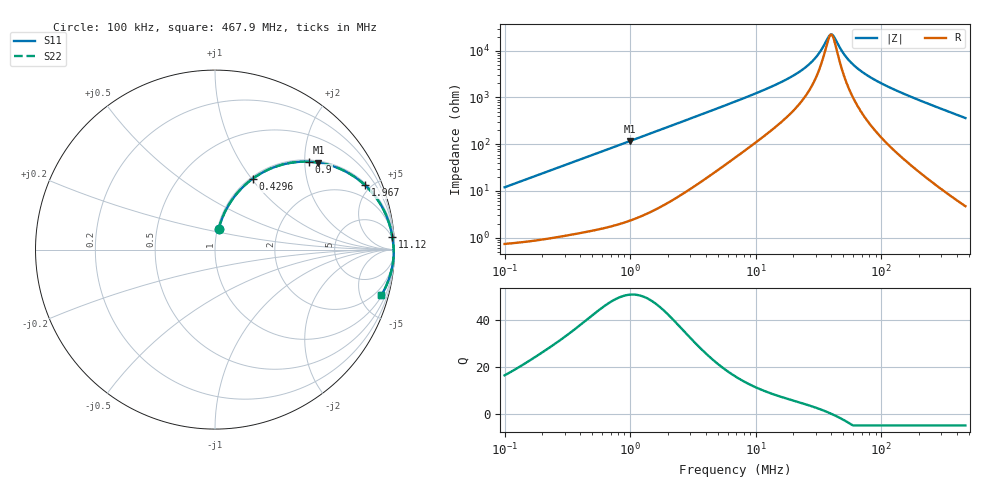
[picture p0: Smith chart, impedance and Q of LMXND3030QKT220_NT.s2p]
! LMXND3030QKT220_NT  S-PARAMETER MODEL  ( Standard Model )
! Model Generated by TAIYO YUDEN Corporation (https://www.yuden.co.jp/en/)
! Version 1.0
! TAIYO YUDEN Control No. 20250724
! Copyright(c) 2025 TAIYO YUDEN CO.,LTD. All Rights Reserved.
! Product Description (link to TY-COMPAS)
! https://ds.yuden.co.jp/TYCOMPAS/or/detail?pn=LMXND3030QKT220MNT&u=M
! Products Name : Inductors
! Characteristics :
!  Inductance : 22 [uH] , SRF(min) : 20 [MHz] , DC Resistance(max) : 0.624 [Ohm]
!  Rated Current : Saturation  470 [m A] , Temp Rise  720 [m A] (40 [degC])
!  Case Size : 3.0 x 3.0 / 0.118 x 0.118 [mm/inch] , Thickness : 1.5 / 0.059 [mm/inch]
!  (Conditions: Temperature = 25 [degC] , DC Bias Current = 0 [A])
! External Node Assignments :
!  1  o---GGG---o  2
! GND o---------o GND
! Frequency Range : 0.1MHz  -  467.920999MHz  [ 402 STEP ]
# MHz S RI R 50
! Freq[MHz].  S11 Real  S11 Imag  S21 Real  S21 Imag  S12 Real  S12 Imag  S22 Real  S22 Imag
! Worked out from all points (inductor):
!   401 points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, 100 kHz to 467.9 MHz, reference 50 ohm
!   read as one part in series: L = 18.9 uH near 104.3 kHz
!   highest Q = 50.6 at 1 MHz (marker M1), where L = 18.6 uH
!   self-resonance near 39.5 MHz
!   S11 on the Smith chart (normalised r, x): 100 kHz: 1.01, +0.24; 429.6 kHz: 1.03, +1.01; 900 kHz: 1.04, +2.11; 1.967 MHz: 1.11, +4.60; 11.12 MHz: 4, +27; 467.9 MHz: 1.09, -7.27
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0.1  0.0209 0.1157  0.9791 -0.1157  0.9791 -0.1157  0.0209 0.1157
0.227951  0.0753 0.2467  0.9247 -0.2467  0.9247 -0.2467  0.0753 0.2467
0.411864  0.1961 0.3842  0.8039 -0.3842  0.8039 -0.3842  0.1961 0.3842
0.42964  0.2091 0.394  0.7909 -0.394  0.7909 -0.394  0.2091 0.394
0.900005  0.5254 0.4895  0.4746 -0.4895  0.4746 -0.4895  0.5254 0.4895
1.000281  0.5765 0.4843  0.4235 -0.4843  0.4235 -0.4843  0.5765 0.4843
1.69632  0.7923 0.3949  0.2077 -0.3949  0.2077 -0.3949  0.7923 0.3949
1.96669  0.8354 0.3593  0.1646 -0.3593  0.1646 -0.3593  0.8354 0.3593
3.335198  0.9318 0.2359  0.0682 -0.2359  0.0682 -0.2359  0.9318 0.2359
6.986533  0.9786 0.1162  0.0214 -0.1162  0.0214 -0.1162  0.9786 0.1162
11.12042  0.9879 0.0708  0.0121 -0.0708  0.0121 -0.0708  0.9879 0.0708
19.67242  0.9929 0.0337  0.00714 -0.0337  0.00714 -0.0337  0.9929 0.0337
28.17346  0.9946 0.0159  0.00542 -0.0159  0.00542 -0.0159  0.9946 0.0159
32.66391  0.9951 0.00904  0.00492 -0.00904  0.00492 -0.00904  0.9951 0.00904
37.87008  0.9955 0.00231  0.00454 -0.00231  0.00454 -0.00231  0.9955 0.00231
40.34804  0.9956 -0.000578  0.00441 0.000578  0.00441 0.000578  0.9956 -0.000578
42.08946  0.9957 -0.00251  0.00434 0.00251  0.00434 0.00251  0.9957 -0.00251
51.99094  0.9958 -0.0124  0.00415 0.0124  0.00415 0.0124  0.9958 -0.0124
61.56461  0.9958 -0.0208  0.00422 0.0208  0.00422 0.0208  0.9958 -0.0208
81.02364  0.9952 -0.0358  0.00483 0.0358  0.00483 0.0358  0.9952 -0.0358
116.0364  0.993 -0.0598  0.00695 0.0598  0.00695 0.0598  0.993 -0.0598
467.921  0.9269 -0.254  0.0731 0.254  0.0731 0.254  0.9269 -0.254
